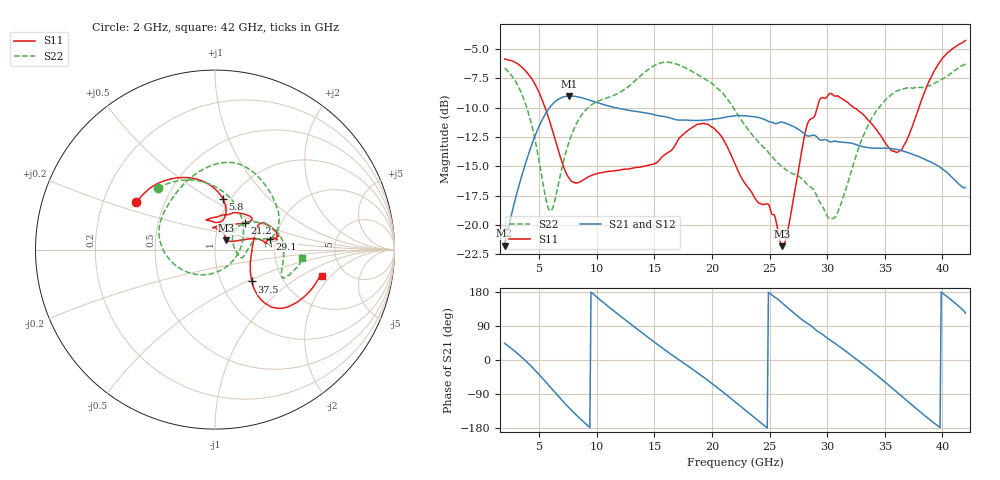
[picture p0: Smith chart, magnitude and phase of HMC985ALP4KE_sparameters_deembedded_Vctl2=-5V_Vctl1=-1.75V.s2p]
!s2p File: Measurements: S11, S21, S12, S22
# GHz S dB R 50.0
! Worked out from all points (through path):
!   401 points, 2 GHz to 42 GHz, reference 50 ohm
!   highest |S21| = -9.00 dB at 7.6 GHz (marker M1); lowest = -21.8 dB at 2 GHz (marker M2)
!   lowest |S11| = -21.8 dB at 26.1 GHz (marker M3), VSWR 1.18, Z = 56.3 + j5.89 ohm
!   |S11| at or under -10 dB: 5.515 GHz to 29.14 GHz (23.62 GHz wide, 136 % of centre); 32.33 GHz to 37.96 GHz (5.631 GHz wide, 16 % of centre)
!   |S22| runs from -19.5 to -6.1 dB; largest |S21 - S12| = 0.0004
!   S11 on the Smith chart (normalised r, x): 2 GHz: 0.35, +0.25; 5.8 GHz: 0.92, +0.57; 21.2 GHz: 1.32, +0.41; 29.1 GHz: 1.86, +0.25; 37.5 GHz: 1.40, -0.54; 42 GHz: 3.34, -1.60
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2  -5.83 148.9  -21.77 44.0  -21.78 44.0  -6.61 132.9
3.2  -6.29 129.7  -16.81 15.1  -16.82 15.1  -8.21 101.8
4.4  -7.59 107.5  -13.04 -19.3  -13.04 -19.3  -11.67 60.9
5.8  -10.81 81.3  -10.13 -65.9  -10.14 -65.9  -18.60 -32.5
7.6  -16.04 78.7  -9.00 -126.2  -9.00 -126.3  -12.89 -154.0
8.7  -16.25 92.5  -9.15 -159.0  -9.15 -159.0  -10.59 177.4
10.2  -15.58 102.0  -9.61 161.1  -9.61 161.1  -9.40 155.1
12.1  -15.31 106.4  -10.10 114.7  -10.10 114.7  -8.63 130.8
15.4  -14.51 82.9  -10.70 38.3  -10.70 38.3  -6.22 83.4
18.2  -11.74 49.2  -11.08 -21.9  -11.09 -21.9  -6.86 51.3
21.2  -13.09 41.7  -10.80 -90.5  -10.80 -90.5  -9.10 15.4
22  -14.79 51.6  -10.69 -110.4  -10.70 -110.4  -10.21 12.1
24.1  -18.17 92.6  -10.85 -162.1  -10.86 -162.1  -13.02 13.6
26.1  -21.83 39.9  -11.24 150.3  -11.25 150.3  -15.04 -3.2
28.7  -10.91 6.9  -12.35 87.9  -12.36 87.9  -16.88 -15.6
29.1  -10.13 11.3  -12.49 77.2  -12.49 77.2  -17.53 -13.2
30.7  -9.02 14.2  -12.85 43.4  -12.86 43.5  -19.35 25.0
33.2  -10.65 30.1  -13.34 -13.7  -13.35 -13.6  -12.26 38.8
35.4  -13.44 7.6  -13.47 -67.8  -13.48 -67.7  -9.04 17.8
37.5  -11.30 -40.7  -14.00 -122.2  -14.01 -122.1  -8.32 -4.8
39.7  -6.20 -41.9  -15.01 -176.0  -15.02 -176.0  -7.72 -22.8
42  -4.25 -14.1  -16.82 123.8  -16.83 123.8  -6.23 -5.4
